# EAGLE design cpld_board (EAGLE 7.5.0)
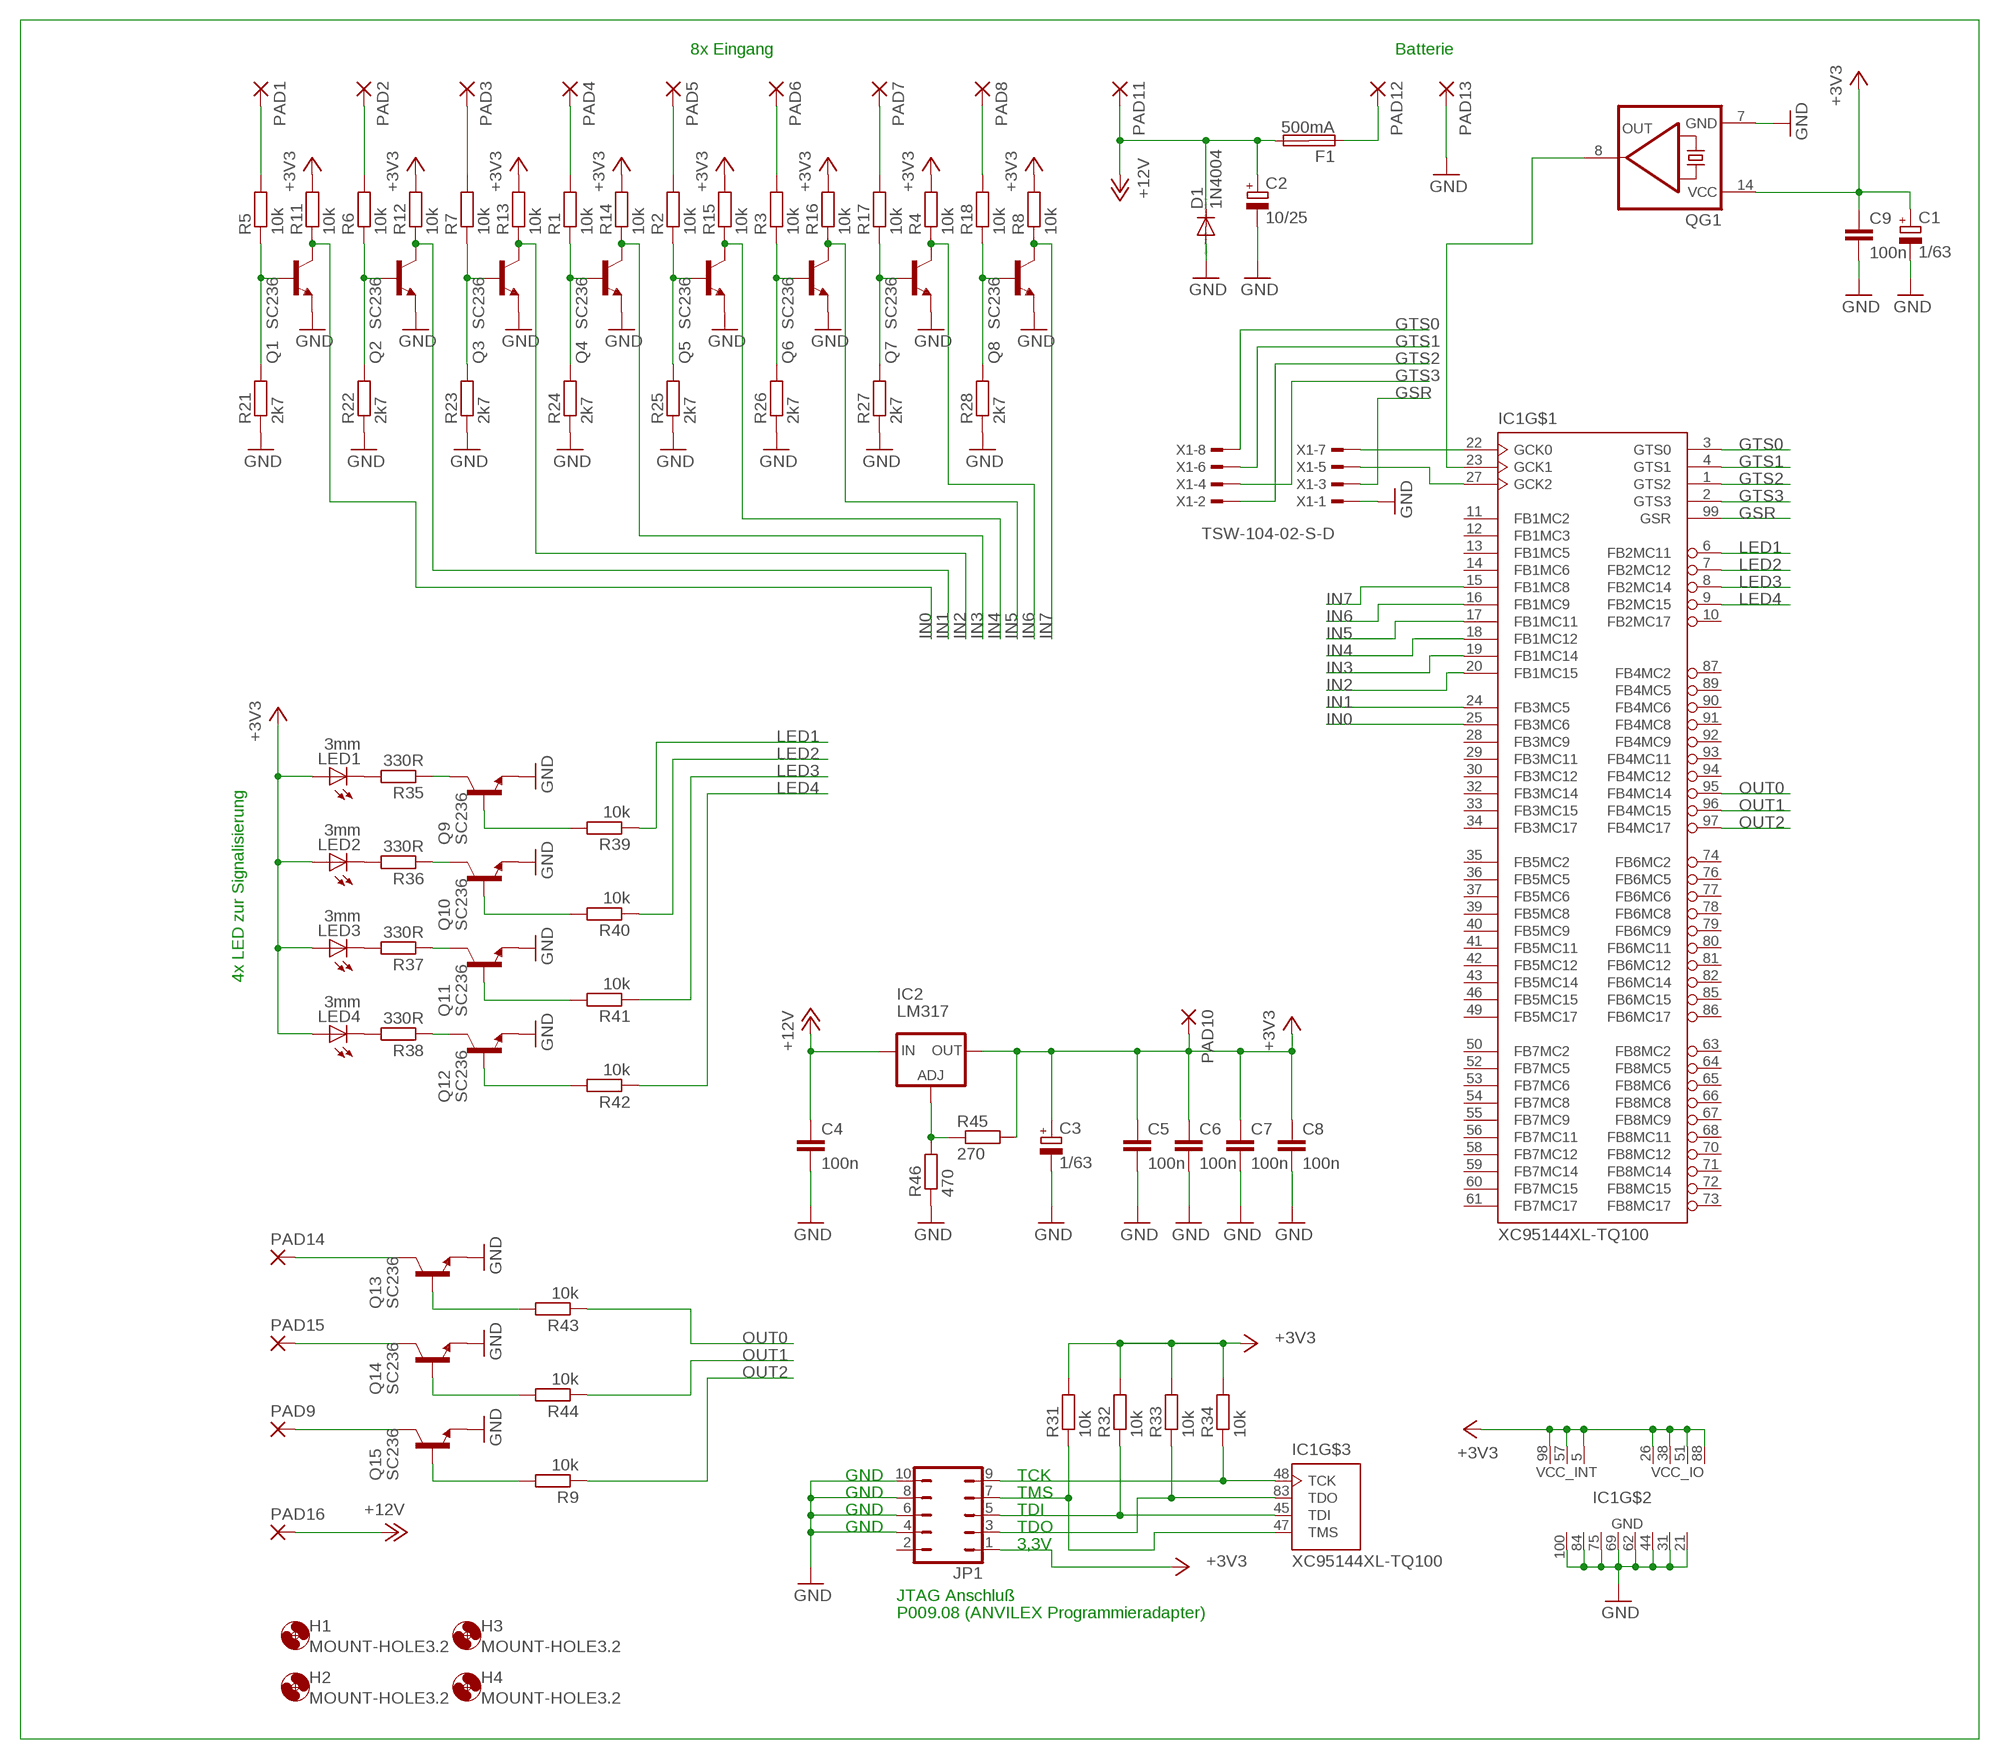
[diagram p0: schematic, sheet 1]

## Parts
C1  1/63  CPOL-EUE2.5-5  [E2,5-5]
C2  10/25  CPOL-EUE2.5-5  [E2,5-5]
C3  1/63  CPOL-EUE2.5-5  [E2,5-5]
C4  100n  C-EU025-025X050  [C025-025X050]
C5  100n  C-EU025-025X050  [C025-025X050]
C6  100n  C-EU025-025X050  [C025-025X050]
C7  100n  C-EU025-025X050  [C025-025X050]
C8  100n  C-EU025-025X050  [C025-025X050]
C9  100n  C-EU025-025X050  [C025-025X050]
D1  1N4004  [DO41-10]
F1  500mA  SHK20L  [SHK20L]
H1  MOUNT-HOLE3.2  [3,2]
H2  MOUNT-HOLE3.2  [3,2]
H3  MOUNT-HOLE3.2  [3,2]
H4  MOUNT-HOLE3.2  [3,2]
IC1  XC95144XL-TQ100  [TQ100]
IC2  LM317  LM317TS  [317TS]
JP1  JP5Q  [JP5Q]
LED1  3mm  LED3MM  [LED3MM]
LED2  3mm  LED3MM  [LED3MM]
LED3  3mm  LED3MM  [LED3MM]
LED4  3mm  LED3MM  [LED3MM]
PAD1  2,15/1,0  [2,15/1,0]
PAD2  2,15/1,0  [2,15/1,0]
PAD3  2,15/1,0  [2,15/1,0]
PAD4  2,15/1,0  [2,15/1,0]
PAD5  2,15/1,0  [2,15/1,0]
PAD6  2,15/1,0  [2,15/1,0]
PAD7  2,15/1,0  [2,15/1,0]
PAD8  2,15/1,0  [2,15/1,0]
PAD9  2,15/1,0  [2,15/1,0]
PAD10  2,15/1,0  [2,15/1,0]
PAD11  2,15/1,0  [2,15/1,0]
PAD12  2,15/1,0  [2,15/1,0]
PAD13  2,15/1,0  [2,15/1,0]
PAD14  2,15/1,0  [2,15/1,0]
PAD15  2,15/1,0  [2,15/1,0]
PAD16  2,15/1,0  [2,15/1,0]
Q1  SC236  BC338  [TO92-EBC]
Q2  SC236  BC338  [TO92-EBC]
Q3  SC236  BC338  [TO92-EBC]
Q4  SC236  BC338  [TO92-EBC]
Q5  SC236  BC338  [TO92-EBC]
Q6  SC236  BC338  [TO92-EBC]
Q7  SC236  BC338  [TO92-EBC]
Q8  SC236  BC338  [TO92-EBC]
Q9  SC236  BC338  [TO92-EBC]
Q10  SC236  BC338  [TO92-EBC]
Q11  SC236  BC338  [TO92-EBC]
Q12  SC236  BC338  [TO92-EBC]
Q13  SC236  BC338  [TO92-EBC]
Q14  SC236  BC338  [TO92-EBC]
Q15  SC236  BC338  [TO92-EBC]
QG1  QG5860  [DIL14S]
R1  10k  R-EU_0207/12  [0207/12]
R2  10k  R-EU_0207/12  [0207/12]
R3  10k  R-EU_0207/12  [0207/12]
R4  10k  R-EU_0207/12  [0207/12]
R5  10k  R-EU_0207/12  [0207/12]
R6  10k  R-EU_0207/12  [0207/12]
R7  10k  R-EU_0207/12  [0207/12]
R8  10k  R-EU_0207/12  [0207/12]
R9  10k  R-EU_0207/12  [0207/12]
R11  10k  R-EU_0207/12  [0207/12]
R12  10k  R-EU_0207/12  [0207/12]
R13  10k  R-EU_0207/12  [0207/12]
R14  10k  R-EU_0207/12  [0207/12]
R15  10k  R-EU_0207/12  [0207/12]
R16  10k  R-EU_0207/12  [0207/12]
R17  10k  R-EU_0207/12  [0207/12]
R18  10k  R-EU_0207/12  [0207/12]
R21  2k7  R-EU_0207/12  [0207/12]
R22  2k7  R-EU_0207/12  [0207/12]
R23  2k7  R-EU_0207/12  [0207/12]
R24  2k7  R-EU_0207/12  [0207/12]
R25  2k7  R-EU_0207/12  [0207/12]
R26  2k7  R-EU_0207/12  [0207/12]
R27  2k7  R-EU_0207/12  [0207/12]
R28  2k7  R-EU_0207/12  [0207/12]
R31  10k  R-EU_0207/12  [0207/12]
R32  10k  R-EU_0207/12  [0207/12]
R33  10k  R-EU_0207/12  [0207/12]
R34  10k  R-EU_0207/12  [0207/12]
R35  330R  R-EU_0207/12  [0207/12]
R36  330R  R-EU_0207/12  [0207/12]
R37  330R  R-EU_0207/12  [0207/12]
R38  330R  R-EU_0207/12  [0207/12]
R39  10k  R-EU_0207/12  [0207/12]
R40  10k  R-EU_0207/12  [0207/12]
R41  10k  R-EU_0207/12  [0207/12]
R42  10k  R-EU_0207/12  [0207/12]
R43  10k  R-EU_0207/12  [0207/12]
R44  10k  R-EU_0207/12  [0207/12]
R45  270  R-EU_0207/12  [0207/12]
R46  470  R-EU_0207/12  [0207/12]
X1  TSW-104-02-S-D  [TSW-104-02-S-D]

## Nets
+3V3: C1.+ C3.+ C5.1 C6.1 C7.1 C8.1 C9.1 IC1.5(VCC_INT) IC1.26(VCC_IO) IC1.38(VCC_IO) IC1.51(VCC_IO) IC1.57(VCC_INT) IC1.88(VCC_IO) IC1.98(VCC_INT) IC2.2(OUT) JP1.1 LED1.A LED2.A LED3.A LED4.A PAD10.1(P) QG1.14(VCC) R4.2 R8.2 R11.2 R12.2 R13.2 R14.2 R15.2 R16.2 R31.2 R32.2 R33.2 R34.2 R45.2
+12V: C2.+ C4.1 D1.C F1.2A IC2.3(IN) PAD11.1(P) PAD16.1(P)
GND: C1.- C2.- C3.- C4.2 C5.2 C6.2 C7.2 C8.2 C9.2 D1.A IC1.21(GND) IC1.31(GND) IC1.44(GND) IC1.62(GND) IC1.69(GND) IC1.75(GND) IC1.84(GND) IC1.100(GND) JP1.4 JP1.6 JP1.8 JP1.10 PAD13.1(P) Q1.E Q2.E Q3.E Q4.E Q5.E Q6.E Q7.E Q8.E Q9.E Q10.E Q11.E Q12.E Q13.E Q14.E Q15.E QG1.7(GND) R21.1 R22.1 R23.1 R24.1 R25.1 R26.1 R27.1 R28.1 R46.1 X1.1
GSR: IC1.99(GSR) X1.3
GTS0: IC1.3(GTS0) X1.8
GTS1: IC1.4(GTS1) X1.6
GTS2: IC1.1(GTS2) X1.2
GTS3: IC1.2(GTS3) X1.4
IN0: IC1.25(FB3MC6) Q1.C R11.1
IN1: IC1.24(FB3MC5) Q2.C R12.1
IN2: IC1.20(FB1MC15) Q3.C R13.1
IN3: IC1.19(FB1MC14) Q4.C R14.1
IN4: IC1.18(FB1MC12) Q5.C R15.1
IN5: IC1.17(FB1MC11) Q6.C R16.1
IN6: IC1.16(FB1MC9) Q7.C R4.1
IN7: IC1.15(FB1MC8) Q8.C R8.1
LED1: IC1.6(FB2MC11) R39.1
LED2: IC1.7(FB2MC12) R40.1
LED3: IC1.8(FB2MC14) R41.1
LED4: IC1.9(FB2MC15) R42.1
N$1: Q9.B R39.2
N$2: IC1.48(TCK) JP1.9 R34.1
N$8: Q1.B R5.1 R21.2
N$9: Q2.B R6.1 R22.2
N$10: Q3.B R7.1 R23.2
N$14: Q4.B R1.1 R24.2
N$15: Q5.B R2.1 R25.2
N$16: Q6.B R3.1 R26.2
N$17: Q7.B R17.1 R27.2
N$18: Q8.B R18.1 R28.2
N$22: PAD8.1(P) R18.2
N$23: PAD7.1(P) R17.2
N$24: PAD6.1(P) R3.2
N$25: PAD5.1(P) R2.2
N$26: PAD4.1(P) R1.2
N$27: PAD3.1(P) R7.2
N$28: PAD2.1(P) R6.2
N$29: PAD1.1(P) R5.2
N$30: PAD9.1(P) Q15.C
N$32: IC1.83(TDO) JP1.3 R33.1
N$33: IC1.47(TMS) JP1.7 R31.1
N$34: IC1.45(TDI) JP1.5 R32.1
N$35: PAD14.1(P) Q13.C
N$36: F1.1A PAD12.1(P)
N$37: LED1.K(C) R35.2
N$38: LED2.K(C) R36.2
N$39: LED4.K(C) R38.2
N$40: LED3.K(C) R37.2
N$41: Q9.C R35.1
N$42: Q10.C R36.1
N$43: Q11.C R37.1
N$44: Q12.C R38.1
N$45: Q15.B R9.2
N$46: Q10.B R40.2
N$47: Q11.B R41.2
N$48: Q12.B R42.2
N$50: IC1.22(GCK0) X1.7
N$53: PAD15.1(P) Q14.C
N$54: Q13.B R43.2
N$55: Q14.B R44.2
N$58: IC1.23(GCK1) QG1.8(OUT)
N$59: IC2.1(ADJ) R45.1 R46.2
N$63: IC1.27(GCK2) X1.5
OUT0: IC1.95(FB4MC14) R43.1
OUT1: IC1.96(FB4MC15) R44.1
OUT2: IC1.97(FB4MC17) R9.1
Unconnected: F1.1B F1.2B IC1.10(FB2MC17) IC1.11(FB1MC2) IC1.12(FB1MC3) IC1.13(FB1MC5) IC1.14(FB1MC6) IC1.28(FB3MC9) IC1.29(FB3MC11) IC1.30(FB3MC12) IC1.32(FB3MC14) IC1.33(FB3MC15) IC1.34(FB3MC17) IC1.35(FB5MC2) IC1.36(FB5MC5) IC1.37(FB5MC6) IC1.39(FB5MC8) IC1.40(FB5MC9) IC1.41(FB5MC11) IC1.42(FB5MC12) IC1.43(FB5MC14) IC1.46(FB5MC15) IC1.49(FB5MC17) IC1.50(FB7MC2) IC1.52(FB7MC5) IC1.53(FB7MC6) IC1.54(FB7MC8) IC1.55(FB7MC9) IC1.56(FB7MC11) IC1.58(FB7MC12) IC1.59(FB7MC14) IC1.60(FB7MC15) IC1.61(FB7MC17) IC1.63(FB8MC2) IC1.64(FB8MC5) IC1.65(FB8MC6) IC1.66(FB8MC8) IC1.67(FB8MC9) IC1.68(FB8MC11) IC1.70(FB8MC12) IC1.71(FB8MC14) IC1.72(FB8MC15) IC1.73(FB8MC17) IC1.74(FB6MC2) IC1.76(FB6MC5) IC1.77(FB6MC6) IC1.78(FB6MC8) IC1.79(FB6MC9) IC1.80(FB6MC11) IC1.81(FB6MC12) IC1.82(FB6MC14) IC1.85(FB6MC15) IC1.86(FB6MC17) IC1.87(FB4MC2) IC1.89(FB4MC5) IC1.90(FB4MC6) IC1.91(FB4MC8) IC1.92(FB4MC9) IC1.93(FB4MC11) IC1.94(FB4MC12) JP1.2

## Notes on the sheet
- 8x Eingang | Batterie
- 4x LED zur Signalisierung
- GND | TCK
- GND | TMS
- GND | TDI
- GND | TDO
- 3,3V
- JTAG Anschluß
- P009.08 (ANVILEX Programmieradapter)

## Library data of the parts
C1-C3 = resistor:CPOL-EU: POLARIZED CAPACITOR, European symbol
C4-C9 = resistor:C-EU: CAPACITOR, European symbol
D1 = diode:1N4004: DIODE
F1 = fuse:SHK20L: FUSE HOLDER 5 x 20 mm, SH contact, SHH1 Schukat, E1073 Buerklin; OC_FARNELL: unknown; OC_NEWARK: unknown
H1-H4 = holes:MOUNT-HOLE: MOUNTING HOLE with drill center marker
IC1 = XC95144XL100:XC95144XL-TQ100
IC2 = v-reg:LM317TS: VOLTAGE REGULATOR
JP1 = jumper:JP5Q: JUMPER
LED1-LED4 = led:LED: LED
PAD1-PAD16 = wirepad:2,15/1,0: THROUGH-HOLE PAD
Q1-Q15 = transistor-npn:BC338*: NPN Transistor
QG1 = crystal:QG5860: CRYSTAL RESONATOR; OC_FARNELL: unknown; OC_NEWARK: unknown
R1-R9 R11-R18 R21-R28 R31-R46 = resistor:R-EU_: RESISTOR, European symbol
X1 = con-samtec:TSW-104-02-S-D: THROUGH-HOLE .025" SQ POST HEADER Source: Samtec TSW.pdf; OC_FARNELL: unknown; OC_NEWARK: unknown

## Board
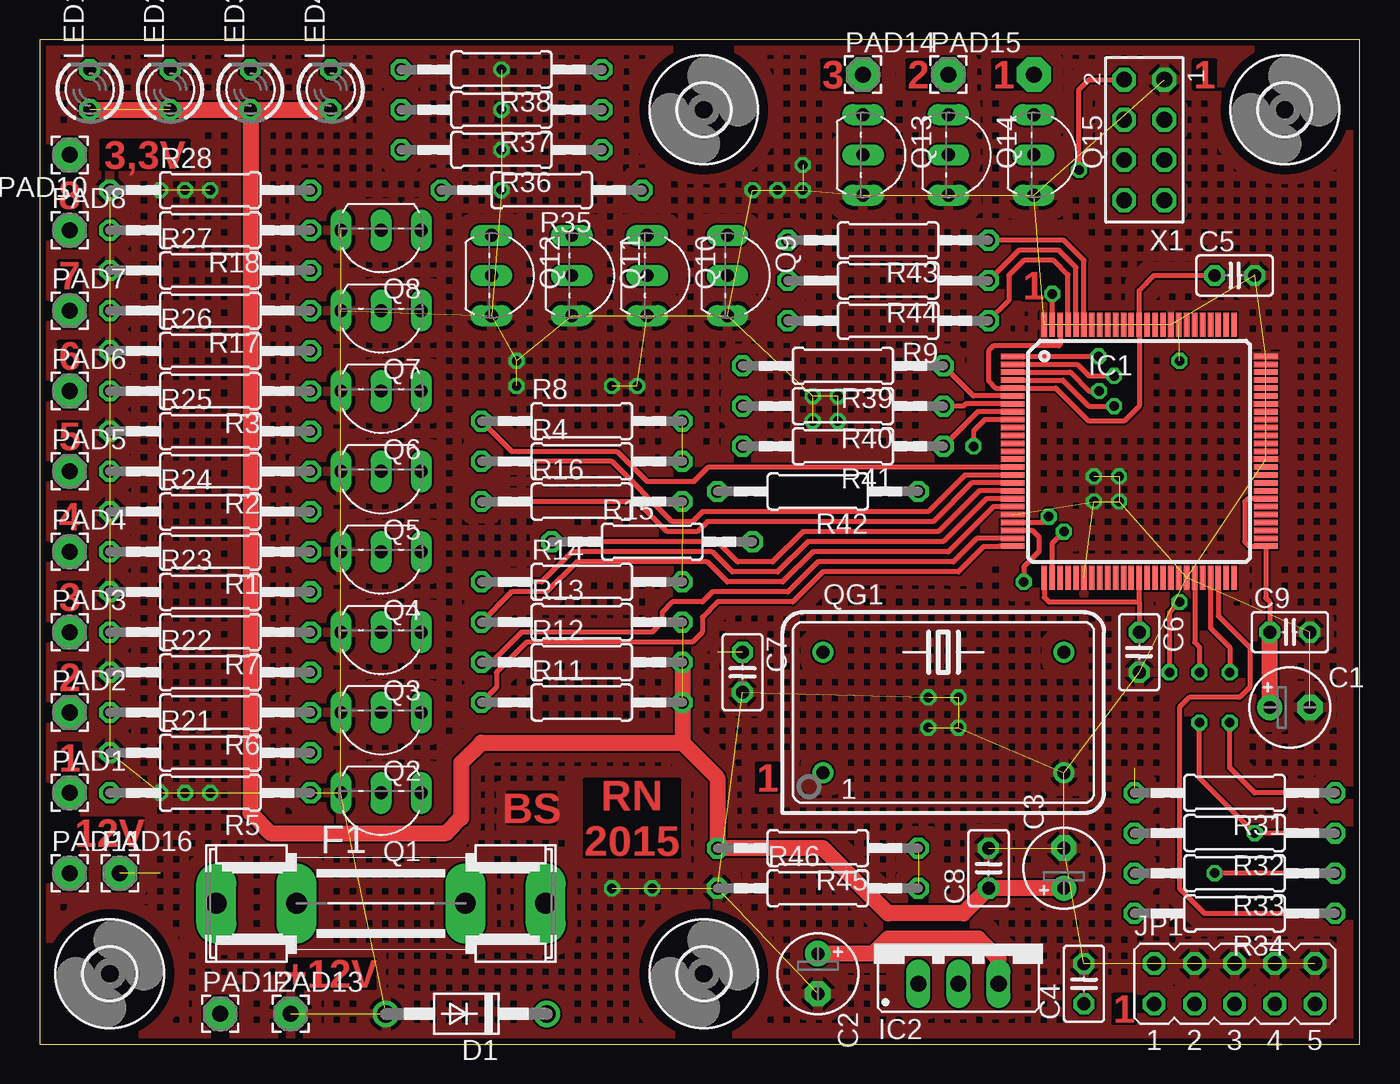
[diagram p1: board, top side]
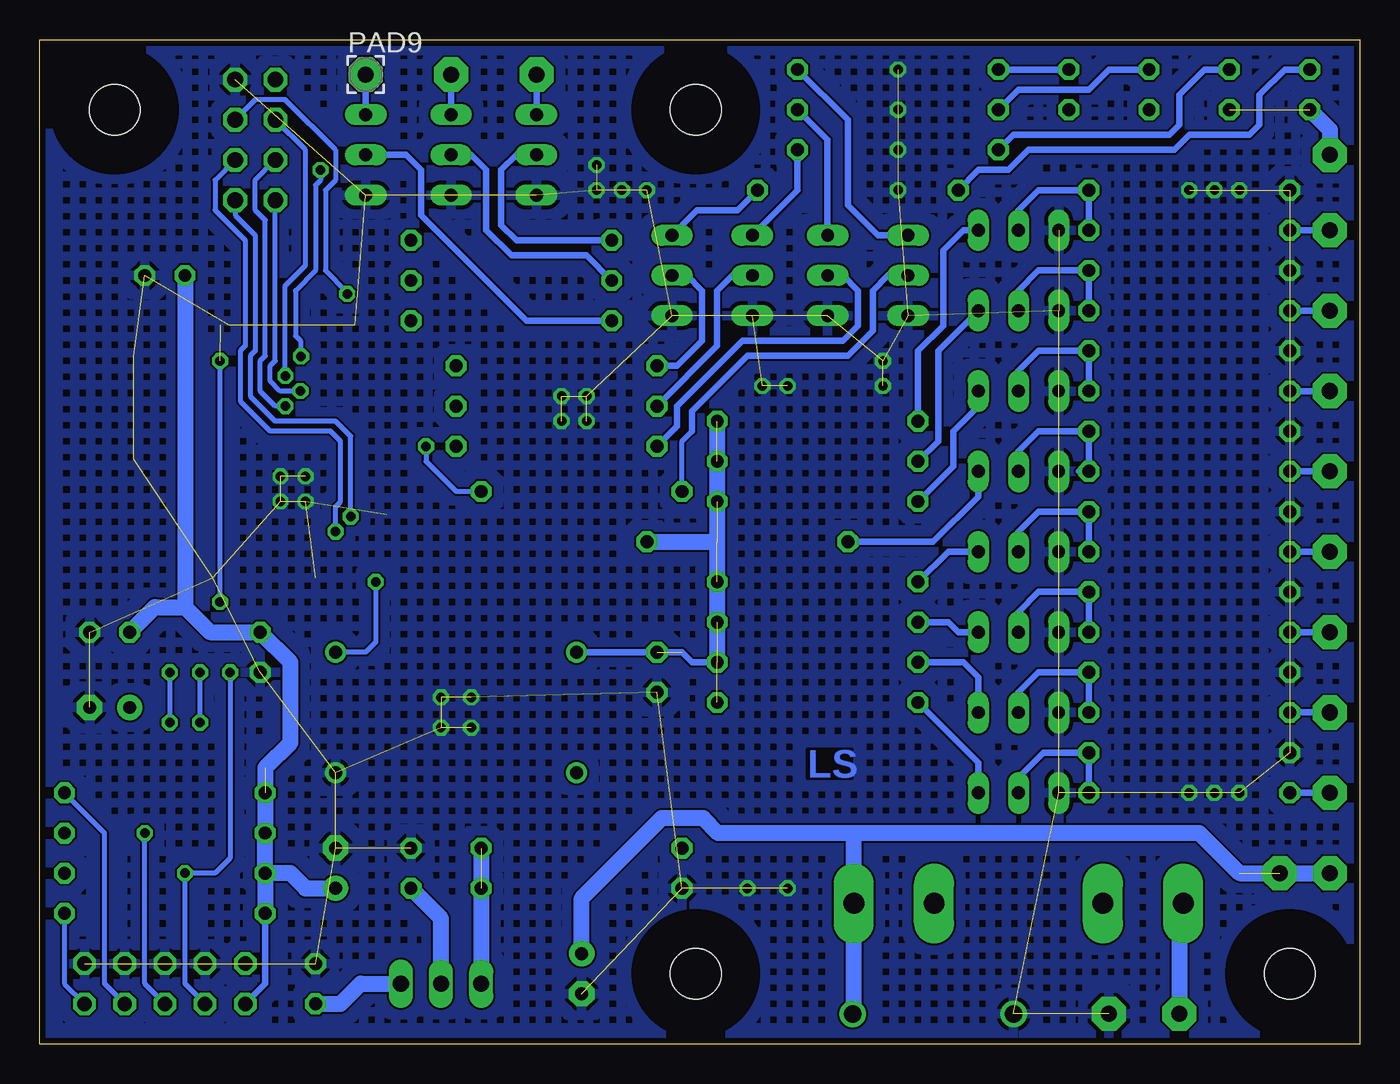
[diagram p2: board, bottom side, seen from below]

Size 83.49 x 63.49 mm. Coordinates in mm from the lower left corner, seen from the top.
Outline: 0,0 83.49,0 83.49,63.49 0,63.49 0,0
Copper layers (1*16): Top 0.035mm / dielectric 1.5mm / Bottom 0.035mm
Design rules "default *": minimum track width 10mil, minimum drill 20mil, track to track 5mil, track to pad 5mil, pad to pad 5mil, via to via 5mil, smd to smd 4mil, copper to edge 15mil, drill to drill 8mil, minimum pad ring 10mil, minimum via ring 8mil, stop-mask expansion 4mil, vias tented up to drill 0mil, thermal gap 10mil

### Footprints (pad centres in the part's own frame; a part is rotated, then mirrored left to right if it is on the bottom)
E2,5-5 = drill 0.813 pad 1.6: + -1.27,0 | drill 0.813 pad 1.6 octagon: - 1.27,0
C025-025X050 = drill 0.813 octagon: 1 -1.27,0; 2 1.27,0
DO41-10 = drill 1.118: A 5.08,0; C -5.08,0
SHK20L = drill 1.321 pad 2.54 long: 1A -10.414,0; 1B -5.334,0; 2A 10.414,0; 2B 5.334,0
3,2 = hole 3.2: 0,0
TQ100 = smd 1.5 x 0.35: 1 -8,6; 2 -8,5.5; 3 -8,5; 4 -8,4.5; 5 -8,4; 6 -8,3.5; 7 -8,3; 8 -8,2.5; 9 -8,2; 10 -8,1.5; 11 -8,1; 12 -8,0.5; 13 -8,0; 14 -8,-0.5; 15 -8,-1; 16 -8,-1.5; 17 -8,-2; 18 -8,-2.5; 19 -8,-3; 20 -8,-3.5; 21 -8,-4; 22 -8,-4.5; 23 -8,-5; 24 -8,-5.5; 25 -8,-6; 51 8,-6; 52 8,-5.5; 53 8,-5; 54 8,-4.5; 55 8,-4; 56 8,-3.5; 57 8,-3; 58 8,-2.5; 59 8,-2; 60 8,-1.5; 61 8,-1; 62 8,-0.5; 63 8,0; 64 8,0.5; 65 8,1; 66 8,1.5; 67 8,2; 68 8,2.5; 69 8,3; 70 8,3.5; 71 8,4; 72 8,4.5; 73 8,5; 74 8,5.5; 75 8,6 | smd 0.35 x 1.5: 26 -6,-8; 27 -5.5,-8; 28 -5,-8; 29 -4.5,-8; 30 -4,-8; 31 -3.5,-8; 32 -3,-8; 33 -2.5,-8; 34 -2,-8; 35 -1.5,-8; 36 -1,-8; 37 -0.5,-8; 38 0,-8; 39 0.5,-8; 40 1,-8; 41 1.5,-8; 42 2,-8; 43 2.5,-8; 44 3,-8; 45 3.5,-8; 46 4,-8; 47 4.5,-8; 48 5,-8; 49 5.5,-8; 50 6,-8; 76 6,8; 77 5.5,8; 78 5,8; 79 4.5,8; 80 4,8; 81 3.5,8; 82 3,8; 83 2.5,8; 84 2,8; 85 1.5,8; 86 1,8; 87 0.5,8; 88 0,8; 89 -0.5,8; 90 -1,8; 91 -1.5,8; 92 -2,8; 93 -2.5,8; 94 -3,8; 95 -3.5,8; 96 -4,8; 97 -4.5,8; 98 -5,8; 99 -5.5,8; 100 -6,8
317TS = drill 1.016 long: 1 -2.54,-2.54; 2 0,-2.54; 3 2.54,-2.54
JP5Q = drill 0.914 octagon: 1 -5.08,-1.27; 2 -5.08,1.27; 3 -2.54,-1.27; 4 -2.54,1.27; 5 0,-1.27; 6 0,1.27; 7 2.54,-1.27; 8 2.54,1.27; 9 5.08,-1.27; 10 5.08,1.27
LED3MM = drill 0.813 octagon: A -1.27,0; K 1.27,0
2,15/1,0 = drill 1.016 pad 2.159 octagon: 1 0,0
TO92-EBC = drill 0.813 long: B 0,-1.27; C -2.54,-1.27; E 2.54,-1.27
DIL14S = drill 0.813: 1 -7.62,-3.81; 7 7.62,-3.81; 8 7.62,3.81; 14 -7.62,3.81
0207/12 = drill 0.813 octagon: 1 -6.35,0; 2 6.35,0
TSW-104-02-S-D = drill 1 pad 1.5 octagon: 1 3.81,-1.27; 2 3.81,1.27; 3 1.27,-1.27; 4 1.27,1.27; 5 -1.27,-1.27; 6 -1.27,1.27; 7 -3.81,-1.27; 8 -3.81,1.27

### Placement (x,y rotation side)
C1  79.06,21.27 0 top
C2  49.21,4.45 270 top
C3  64.77,11.11 90 top
C4  66.04,3.81 90 top
C5  75.56,48.58 0 top
C6  69.53,24.77 270 top
C7  44.45,23.5 270 top
C8  60.01,11.11 90 top
C9  79.06,26.04 0 top
D1  26.99,1.91 180 top
F1  21.59,8.89 0 top
H1  42,4.45 0 top
H2  4.45,4.45 0 top
H3  78.74,59.05 0 top
H4  42,59.05 0 top
IC1  69.53,37.47 0 top
IC2  58.1,6.35 0 top
JP1  75.56,3.81 0 top
LED1  3.17,60.33 90 top
LED2  8.26,60.33 90 top
LED3  13.34,60.33 90 top
LED4  18.41,60.33 90 top
PAD1  1.91,15.88 0 top
PAD2  1.91,20.95 0 top
PAD3  1.91,26.04 0 top
PAD4  1.91,31.11 0 top
PAD5  1.91,36.2 0 top
PAD6  1.91,41.27 0 top
PAD7  1.91,46.35 0 top
PAD8  1.91,51.44 0 top
PAD9  62.87,61.28 0 bottom
PAD10  1.91,56.2 180 top
PAD11  1.91,10.79 0 top
PAD12  11.43,1.91 0 top
PAD13  15.88,1.91 0 top
PAD14  52.07,61.28 0 top
PAD15  57.47,61.28 0 top
PAD16  5.08,10.79 0 top
Q1  21.59,14.61 180 top
Q2  21.59,19.68 180 top
Q3  21.59,24.77 180 top
Q4  21.59,29.84 180 top
Q5  21.59,34.92 180 top
Q6  21.59,40.01 180 top
Q7  21.59,45.09 180 top
Q8  21.59,50.16 180 top
Q9  44.77,48.58 270 top
Q10  39.69,48.58 270 top
Q11  34.92,48.58 270 top
Q12  29.84,48.58 270 top
Q13  53.34,56.2 270 top
Q14  58.74,56.2 270 top
Q15  64.14,56.2 270 top
QG1  57.15,20.95 0 top
R1  10.79,31.11 180 top
R2  10.79,36.2 180 top
R3  10.79,41.27 180 top
R4  34.29,36.83 0 top
R5  10.79,15.88 180 top
R6  10.79,20.95 180 top
R7  10.79,26.04 180 top
R8  34.29,39.37 0 top
R9  53.66,45.72 180 top
R11  34.29,21.59 0 top
R12  34.29,24.13 0 top
R13  34.29,26.67 0 top
R14  34.29,29.21 0 top
R15  38.73,31.75 0 top
R16  34.29,34.29 0 top
R17  10.79,46.35 180 top
R18  10.79,51.44 180 top
R21  10.79,18.41 0 top
R22  10.79,23.5 0 top
R23  10.79,28.57 0 top
R24  10.79,33.66 0 top
R25  10.79,38.73 0 top
R26  10.79,43.81 0 top
R27  10.79,48.9 0 top
R28  10.79,53.98 0 top
R31  75.56,15.88 180 top
R32  75.56,13.34 180 top
R33  75.56,10.79 180 top
R34  75.56,8.26 180 top
R35  31.75,53.98 180 top
R36  29.21,56.52 180 top
R37  29.21,59.05 180 top
R38  29.21,61.59 180 top
R39  50.8,42.86 180 top
R40  50.8,40.32 180 top
R41  50.8,37.78 180 top
R42  49.21,34.92 180 top
R43  53.66,50.8 180 top
R44  53.66,48.26 180 top
R45  49.21,12.38 180 top
R46  49.21,9.84 0 top
X1  69.85,57.15 90 top

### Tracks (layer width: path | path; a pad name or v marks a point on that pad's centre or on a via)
+3V3  (8 unrouted)
  Top 0.305: IC1.98 64.53,44.21 64.45,44.13 60.33,44.13 60.01,43.81 60.01,41.91 60.45,41.47 IC1.5 64.26,41.47 66.36,39.37 68.58,39.37 69.53,40.32 IC1.88 69.53,47.62 70.48,48.58 C5.1 | IC1.26 63.53,28.23 63.82,27.94 69.53,27.94 | 69.53,27.94 IC1.38 | C9.1 77.79,27.94 77.53,28.2 IC1.51 76.48,31.46 76.2,31.75 76.2,34.29 76.38,34.47 IC1.57 | 69.53,27.94 C6.1
  Top 1.016: LED1.A LED3.A | LED3.A LED4.A | LED3.A 13.34,14.61 14.61,13.34 25.72,13.34 26.67,14.29 26.67,17.78 27.94,19.05 40.64,19.05 | C1.+ C9.1 | R12.2 40.64,19.05 | 40.64,19.05 42.86,16.83 R45.2 49.53,12.38 53.66,8.26 58.42,8.26 C8.1 C3.+
  Bottom 0.406: R12.2 42.23,24.13 42.86,24.77 QG1.14 | R34.2 69.22,3.81 JP1.1
  Bottom 1.016: R33.2 R34.2 | LED1.A 1.91,57.78 PAD10.1 | R33.2 67.63,10.79 66.67,9.84 C3.+ | R8.2 40.64,31.75 | 40.64,31.75 R12.2 | R15.2 40.64,31.75 | R33.2 R32.2 69.22,17.46 67.63,19.05 67.63,24.13 C6.1 72.71,26.04 74.3,27.62 | C9.1 76.2,27.62 74.3,27.62 | IC2.2 58.1,7.94 C8.1 | C5.1 74.3,27.62
+12V  (1 unrouted)
  Top 1.016: IC2.3 60.64,5.4 59.37,6.67 53.66,6.67 52.7,5.71 C2.+
  Bottom 1.016: 32.07,13.34 10.16,13.34 7.62,10.79 PAD11.1 | 32.07,13.34 40.58,13.34 41.53,14.29 44.13,14.29 49.21,9.21 C2.+ | C4.1 64.45,2.54 63.18,3.81 IC2.3 | 32.07,13.34 arc90 32,13.27 F1.2A 32,1.91 D1.C
GND  (via drill 0.6)  (80 unrouted)
  other vias: 66.67,35.88 66.67,34.29 68.26,35.88 68.26,34.29 29.21,59.05 29.21,56.52 29.21,61.59 29.21,53.98 30.16,41.59 37.78,41.59 45.09,53.98 48.26,55.56 46.67,53.98 48.26,53.98 48.9,40.96 50.48,40.96 48.9,39.37 50.48,39.37 56.2,21.91 56.2,20 58.1,20 58.1,21.91 36.2,9.84 38.73,9.84 7.62,15.88 10.79,15.88 9.21,15.88 10.79,53.98 7.62,53.98 9.21,53.98 30.16,43.18 36.2,41.59
  pour Top (hatched): 0,63.5 83.82,63.5 83.82,0 0,0
  pour Bottom (hatched): 0,63.5 83.82,63.5 83.82,46.99 83.82,0 0,0
GSR  (via drill 0.6)
  Top 0.305: IC1.99 v64.03,47.41
  Bottom 0.305: v64.03,47.41 64.03,47.52 65.41,48.9 65.41,53.98 64.77,54.61 64.77,56.52 67.94,59.69 69.85,59.69 X1.3
GTS0  (via drill 0.6)
  Top 0.305: IC1.3 65.17,42.47 66.36,41.27 v66.99,41.27
  Bottom 0.305: v66.99,41.27 68.26,41.27 68.9,41.91 68.9,42.86 68.58,43.18 X1.8
GTS1  (via drill 0.6)
  Top 0.305: IC1.4 64.72,41.97 66.36,40.32 v67.94,40.32
  Bottom 0.305: v67.94,40.32 68.58,40.32 69.53,41.27 69.53,43.18 69.22,43.5 69.22,52.07 69.85,52.7 69.85,54.61 X1.6
GTS2  (via drill 0.6)
  Top 0.305: IC1.1 v66.96,43.47 | v65.72,55.24 65.72,60.33 66.36,60.96 X1.2
  Bottom 0.305: v65.72,55.24 65.72,54.61 66.04,54.29 66.04,48.9 67.31,47.62 67.31,44.77 66.99,44.45 66.99,43.5 v66.96,43.47
GTS3  (via drill 0.6)
  Top 0.305: IC1.2 65.62,42.97 66.36,42.23 v67.94,42.23
  Bottom 0.305: v67.94,42.23 67.94,47.94 66.67,49.21 66.67,56.52 X1.4
IN0
  Top 0.305: IC1.25 60.67,31.46 60.64,31.43 59.69,31.43 58.1,29.84 49.53,29.84 47.62,27.94 42.86,27.94 41.91,26.99 41.91,26.04 41.27,25.4 30.8,25.4 28.89,23.5 28.89,22.54 R11.1
  Bottom 0.406: R11.1 24.13,17.78 Q1.C
IN1
  Top 0.305: IC1.24 59.27,31.96 57.78,30.48 49.21,30.48 47.31,28.57 42.55,28.57 41.91,27.94 40.01,27.94 39.37,27.3 39.37,26.67 38.73,26.04 30.48,26.04 28.57,24.13 R12.1
  Bottom 0.406: R12.1 25.08,24.13 24.13,23.18 Q2.C
IN2
  Top 0.305: IC1.20 60.32,33.97 57.47,31.11 48.9,31.11 46.99,29.21 43.5,29.21 42.23,30.48 33.97,30.48 32.07,28.57 29.84,28.57 R13.1
  Bottom 0.406: Q3.C 25.4,26.04 26.04,26.67 R13.1
IN3
  Top 0.305: IC1.19 59.87,34.47 57.15,31.75 48.58,31.75 46.67,29.84 43.81,29.84 42.55,31.11 33.66,31.11 31.75,29.21 R14.1
  Bottom 0.406: Q4.C 26.04,31.11 R14.1
IN4
  Top 0.305: IC1.18 59.41,34.97 56.83,32.38 48.26,32.38 46.35,30.48 44.13,30.48 42.86,31.75 R15.1
  Bottom 0.406: Q5.C 24.13,34.61 26.99,31.75 R15.1
IN5
  Top 0.305: IC1.17 58.96,35.47 56.52,33.02 42.23,33.02 41.59,32.38 39.69,32.38 37.78,34.29 R16.1
  Bottom 0.406: R16.1 25.72,36.51 25.72,38.73 24.13,40.32 Q6.C
IN6
  Top 0.305: IC1.16 58.51,35.97 56.2,33.66 41.91,33.66 41.27,33.02 40.01,33.02 36.2,36.83 R4.1
  Bottom 0.406: Q7.C 26.67,43.81 26.67,38.1 R4.1
IN7
  Top 0.305: R8.1 29.84,37.47 36.51,37.47 38.42,35.56 41.37,35.56 42.27,36.47 IC1.15
  Bottom 0.406: Q8.C 25.08,51.44 26.35,50.16 26.35,45.4 27.94,43.81 R8.1
LED1
  Top 0.305: IC1.6 59.05,40.97 R39.1
LED2
  Top 0.305: IC1.7 58.56,40.47 58.42,40.32 R40.1
LED3
  Top 0.305: IC1.8 59.33,39.97 R41.1
LED4  (via drill 0.6)
  Top 0.305: IC1.9 59.78,39.47 59.05,38.73 v59.05,37.78
  Bottom 0.305: v59.05,37.78 59.05,36.83 57.15,34.92 R42.1
N$1
  Bottom 0.406: R39.2 43.18,42.86 41.59,44.45 41.59,47.62 42.55,48.58 Q9.B
N$2
  Top 0.305: IC1.48 74.53,27.07 76.52,25.08 76.52,22.54 75.88,21.91 72.71,21.91 72.07,21.27 72.07,9.84 73.66,8.26 R34.1
  Bottom 0.305: R34.1 81.92,3.81 JP1.9
N$8
  Bottom 0.406: R5.1 R21.2 20,18.41 21.59,16.83 Q1.B
N$9
  Bottom 0.406: R6.1 R22.2 20.32,23.5 21.59,22.23 Q2.B
N$10
  Bottom 0.406: R7.1 R23.2 20.32,28.57 21.59,27.3 Q3.B
N$14
  Bottom 0.406: R1.1 R24.2 20.32,33.66 21.59,32.38 Q4.B
N$15
  Bottom 0.406: 17.78,36.2 R2.1 R25.2 20.32,38.73 21.59,37.47 Q5.B
N$16
  Bottom 0.406: R3.1 R26.2 20.32,43.81 21.59,42.55 Q6.B
N$17
  Bottom 0.406: R17.1 R27.2 20.32,48.9 21.59,47.62 Q7.B
N$18
  Bottom 0.406: R18.1 R28.2 20.32,53.98 21.59,52.7 Q8.B
N$22
  Bottom 0.406: PAD8.1 R18.2
N$23
  Bottom 0.406: PAD7.1 R17.2
N$24
  Bottom 0.406: PAD6.1 R3.2
N$25
  Bottom 0.406: PAD5.1 R2.2
N$26
  Bottom 0.406: PAD4.1 R1.2
N$27
  Bottom 0.406: PAD3.1 R7.2
N$28
  Bottom 0.406: PAD2.1 R6.2
N$29
  Bottom 0.406: PAD1.1 R5.2
N$30
  Bottom 0.406: PAD9.1 Q15.C
N$32  (via drill 0.6)  (1 unrouted)
  Top 0.305: R33.1 v74.3,10.79 | v72.07,27.94 71.44,27.3 v71.44,23.5
  Bottom 0.305: v72.07,27.94 v72.07,43.18 | v71.44,23.5 71.44,11.75 72.39,10.79 v74.3,10.79 74.3,3.81 JP1.3
N$33  (via drill 0.6)
  Top 0.305: IC1.47 74.03,26.3 75.25,25.08 v75.25,23.5 | R31.1 76.83,15.88 75.25,17.46 v75.25,20.32
  Bottom 0.305: v75.25,23.5 v75.25,20.32 | JP1.7 79.38,3.81 79.38,13.34 R31.1
N$34  (via drill 0.6)
  Top 0.305: IC1.45 73.03,25.39 73.34,25.08 v73.34,23.5 | R32.1 v76.83,13.34 73.34,16.83 v73.34,20.32
  Bottom 0.305: JP1.5 76.83,3.81 v76.83,13.34 | v73.34,20.32 v73.34,23.5
N$35
  Bottom 0.406: Q13.C PAD14.1
N$36
  Bottom 1.016: F1.1A 11.43,8.64 PAD12.1
N$37
  Bottom 0.406: R35.2 24.13,55.24 22.23,55.24 20.95,56.52 11.75,56.52 10.79,57.47 6.99,57.47 6.35,58.1 6.35,60.01 4.76,61.59 LED1.K
N$38
  Bottom 0.406: R36.2 21.91,57.47 12.06,57.47 11.43,58.1 11.43,60.01 9.84,61.59 LED2.K
N$39
  Bottom 0.406: R38.2 LED4.K
N$40
  Bottom 0.406: R37.2 21.59,60.33 17.14,60.33 15.88,61.59 LED3.K
N$41
  Bottom 0.406: R35.1 39.37,52.7 41.91,52.7 Q9.C
N$42
  Bottom 0.406: R36.1 35.56,53.98 Q10.C
N$43
  Bottom 0.406: R37.1 33.66,57.15 Q11.C
N$44
  Bottom 0.406: R38.1 32.38,58.42 32.38,53.02 30.48,51.12 Q12.C
N$45
  Bottom 0.406: Q15.B 60.33,56.2 59.37,55.24 59.37,52.39 52.7,45.72 R9.2
N$46
  Bottom 0.406: Q10.B 39.69,48.58 40.64,47.62 40.64,44.13 R40.2
N$47
  Bottom 0.406: R41.2 43.18,39.05 43.18,40.32 39.05,44.45 32.7,44.45 31.75,45.4 31.75,47.62 32.7,48.58 Q11.B
N$48
  Bottom 0.305: R42.2 42.86,38.1 42.23,38.73
  Bottom 0.406: Q12.B 29.84,48.58 30.8,47.62 30.8,45.09 32.38,43.5 38.73,43.5 42.23,40.01 42.23,38.73
N$50  (via drill 0.6)
  Top 0.305: IC1.22 63.45,32.97 v63.82,33.34
  Bottom 0.305: X1.7 71.12,52.39 69.85,51.12 69.85,43.81 70.17,43.5 70.17,40.96 68.58,39.37 64.77,39.37 63.82,38.42 v63.82,33.34
N$53
  Bottom 0.406: PAD15.1 Q14.C
N$54
  Bottom 0.406: R43.2 53.34,50.8 54.29,51.75 54.29,55.24 53.34,56.2 Q13.B
N$55
  Bottom 0.406: Q14.B 56.2,56.2 55.24,55.24 55.24,51.44 53.66,49.85 48.9,49.85 R44.2
N$58  (via drill 0.6)
  Top 0.305: IC1.23 62.78,32.47 63.18,32.07 63.18,31.11 62.23,30.16 v62.23,29.21
  Bottom 0.305: v62.23,29.21 62.23,25.4 62.87,24.77 QG1.8
N$59  (1 unrouted)
  Bottom 1.016: R45.1 IC2.1
N$63  (via drill 0.6)
  Top 0.305: IC1.27 64.03,31.65 v64.77,32.38
  Bottom 0.305: X1.5 72.39,54.61 72.39,52.7 70.48,50.8 70.48,44.13 70.8,43.81 70.8,40.64 68.9,38.73 65.09,38.73 64.45,38.1 64.45,34.29 64.77,33.97 v64.77,32.38
OUT0
  Top 0.305: IC1.95 66.03,49.54 64.77,50.8 R43.1
OUT1
  Top 0.305: IC1.96 65.53,49.09 64.45,50.16 61.91,50.16 R44.1
OUT2
  Top 0.305: IC1.97 65.03,48.63 64.14,49.53 62.23,49.53 61.28,48.58 61.28,46.99 R9.1

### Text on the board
Top: 3 | 2 | 1 | 1 | 3,3V | 8 | 7 | 1 | 6 | 5 | 4 | 3 | 2 | 1 | 1 | BS | RN / 2015 | 12V | +12V | 1
Bottom: LS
